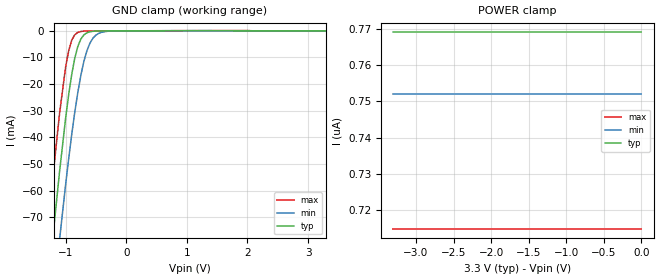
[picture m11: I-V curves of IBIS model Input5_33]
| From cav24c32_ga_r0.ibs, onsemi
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|//////////////////////////////////////////////////////////////////////////////
|//////////////////////////////////////////////////////////////////////////////
[Model]  Input5_33
Model_type Input
Vinh = 2.31
Vinl = 0.99
|  variable   typ   min   max
C_comp   6pF   6pF   6pF
|//////////////////////////////////////////////////////////////////////////////
[Temperature Range]   25   125   -40
|//////////////////////////////////////////////////////////////////////////////
[Voltage Range]   3.30V   3.00V   3.60V
|//////////////////////////////////////////////////////////////////////////////
[POWER Clamp Reference] 3.30V   3.00V   3.60V
|//////////////////////////////////////////////////////////////////////////////
[GND Clamp Reference]   0V   0V   0V
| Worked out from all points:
|   GND clamp passes 1 mA (typ) near -0.67 V on its own axis
|//////////////////////////////////////////////////////////////////////////////
[GND Clamp]
|   Voltage   I(typ)   I(min)   I(max)
-3.3V     -636mA     -636mA     -626mA
-1.3V     -98.7mA    -123mA     -76.2mA
-1.2V     -75mA      -100mA     -52.5mA
-1.1V     -52.7mA    -78.2mA    -30.9mA
-1V       -32.7mA    -57.6mA    -13.5mA
-950mV    -23.9mA    -48mA      -7.46mA
-900mV    -16.4mA    -38.9mA    -3.54mA
-800mV    -5.92mA    -23.2mA    -602uA
-700mV    -1.53mA    -11.5mA    -125uA
-600mV    -354uA     -4.66mA    -56uA
-400mV    -38.7uA    -506uA     -31uA
3.3V      769nA      752nA      715nA
|//////////////////////////////////////////////////////////////////////////////
[POWER Clamp]
|   Voltage   I(typ)   I(min)   I(max)
-3.3V     769nA      752nA      715nA
-3.2V     769nA      752nA      715nA
-3.1V     769nA      752nA      715nA
0V        769nA      752nA      715nA
